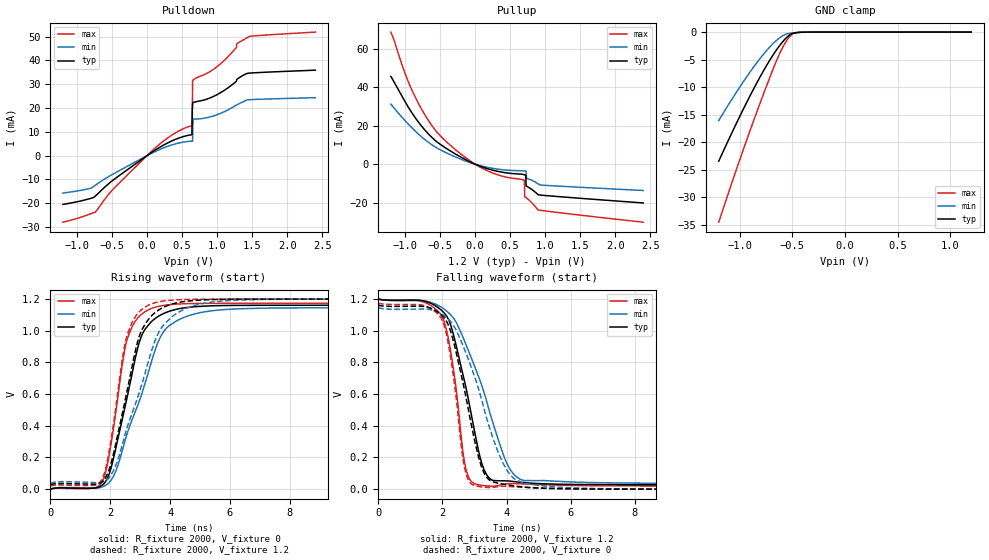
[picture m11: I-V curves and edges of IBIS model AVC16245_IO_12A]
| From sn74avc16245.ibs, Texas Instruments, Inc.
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[Model]   AVC16245_IO_12A
Model_type  I/O
Vinl = 0
Vinh = 1.2
Enable   Active-Low
Vref =   0
Rref =   2000
Cref =   30p
Vmeas =   0.6
| variable   typ   min   max
C_comp   6.68pF   6.18pF   7.38pF
| C_pullup   3.49pF   0.03pF   6.05pF
| C_pulldown   6.30pF   2.05pF   10.38pF
| C_tri-state   6.68pF   6.18pF   7.38pF
[Temperature Range]   40   100   -40
| Ambient temperature   25   85   -40
[Voltage range]   1.2   1.2   1.2
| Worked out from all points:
|   slope of the pulldown table from 0 to 0.18 V, typ, clamps not added: 51.7 ohm
|   slope of the pullup table from 0 to 0.18 V, typ, clamps not added: 75.9 ohm
|   GND clamp passes 1 mA (typ) near -0.56 V on its own axis
|   rising waveform, R_fixture 2000, V_fixture 0: 20-80 % time 818ps typ, 1.19ns min, 574ps max; typ from 0 V to 1.16 V
|   falling waveform, R_fixture 2000, V_fixture 1.2: 20-80 % time 749ps typ, 1.19ns min, 455ps max; typ from 1.2 V to 0.028 V
|   rising waveform, R_fixture 2000, V_fixture 1.2: 20-80 % time 816ps typ, 1.18ns min, 575ps max; typ from 0.028 V to 1.2 V
|   falling waveform, R_fixture 2000, V_fixture 0: 20-80 % time 741ps typ, 1.13ns min, 445ps max; typ from 1.16 V to 0 V
[GND Clamp]
| AVC16245_IO_12A
|   Voltage   I(typ)   I(min)   I(max)
-1.2V     -23.48mA   -16.09mA   -34.58mA
-1.055V   -17.52mA   -11.63mA   -26.28mA
-920mV    -12.26mA   -7.746mA   -18.87mA
-800mV    -7.914mA   -4.632mA   -12.58mA
-700mV    -4.663mA   -2.414mA   -7.551mA
-640mV    -2.948mA   -1.337mA   -4.735mA
-590mV    -1.713mA   -656.6uA   -2.719mA
-545mV    -820.2uA   -290.5uA   -1.288mA
-505mV    -294.5uA   -174.3uA   -438.8uA
-455mV    -91.21uA   -79.33uA   -93.44uA
-385mV    -13.73uA   -21.91uA   -7.311uA
1.2V      671.7pA    3.121nA    23.8pA
[Pulldown]
| AVC16245_IO_12A
|   Voltage   I(typ)   I(min)   I(max)
-1.2V     -20.49mA   -15.71mA   -27.96mA
-735mV    -16.93mA   -12.4mA    -23.63mA
-490mV    -10.42mA   -7.841mA   -14.3mA
105mV     2.117mA    1.578mA    2.919mA
640mV     8.777mA    6.078mA    12.49mA
645mV     19.09mA    6.084mA    12.56mA
650mV     22.11mA    6.1mA      31.26mA
655mV     22.27mA    14.99mA    31.78mA
1.02V     25.96mA    17.43mA    37.88mA
1.29V     32.23mA    21.49mA    47.14mA
1.46V     34.67mA    23.51mA    50.08mA
2.4V      35.9mA     24.35mA    51.89mA
[Pullup]
| AVC16245_IO_12A
|   Voltage   I(typ)   I(min)   I(max)
-1.2V     45.5mA     31.17mA    68.57mA
-950mV    29.56mA    20.73mA    42.76mA
-735mV    18.6mA     13.35mA    26.89mA
-175mV    3.153mA    2.205mA    4.536mA
230mV     -2.893mA   -2.023mA   -4.269mA
705mV     -5.502mA   -3.55mA    -8.484mA
710mV     -5.555mA   -3.566mA   -16.92mA
725mV     -5.74mA    -3.634mA   -17.28mA
730mV     -11.38mA   -3.665mA   -17.41mA
735mV     -11.47mA   -7.353mA   -17.54mA
900mV     -15.81mA   -10.2mA    -23.72mA
2.4V      -20.15mA   -13.67mA   -30.14mA
[Ramp]
| AVC16245_IO_12A
| variable   typ   min   max
dV/dt_r   0.70/8.23E-10   0.69/1.19E-09   0.70/5.77E-10
dV/dt_f   0.70/7.51E-10   0.70/1.19E-09   0.71/4.59E-10
R_load = 2000
[Rising Waveform]
| AVC16245_IO_12A
R_fixture =   2000
C_fixture =   0
L_fixture =   0
V_fixture =   0
V_fixture_min = 0
V_fixture_max = 0
|   Time   V(typ)   V(min)   V(max)
0s        24.7nV     138.2nV    665.8pV
1.51ns    7.743mV    6.93mV     9.912mV
1.845ns   47.28mV    24.35mV    105.5mV
2.18ns    251.3mV    110.4mV    473.7mV
2.605ns   614.7mV    372.8mV    967.2mV
3.08ns    981.3mV    617mV      1.109V
3.865ns   1.115V     1.014V     1.162V
4.995ns   1.154V     1.114V     1.172V
7.165ns   1.161V     1.143V     1.173V
50ns      1.161V     1.145V     1.173V
[Falling Waveform]
| AVC16245_IO_12A
R_fixture =   2000
C_fixture =   0
L_fixture =   0
V_fixture =   1.2
V_fixture_min = 1.2
V_fixture_max = 1.2
|   Time   V(typ)   V(min)   V(max)
0s        1.2V       1.2V       1.2V
1.35ns    1.19V      1.191V     1.185V
1.99ns    1.126V     1.146V     1.089V
2.285ns   1.018V     1.094V     836.7mV
2.74ns    636.1mV    910.6mV    122.6mV
3.27ns    137.7mV    627.6mV    22.9mV
3.53ns    59.43mV    447.8mV    18.77mV
4.005ns   52.17mV    164.8mV    33.91mV
4.58ns    40.67mV    53.88mV    32.26mV
50ns      27.74mV    36.95mV    20.19mV
[Rising Waveform]
| AVC16245_IO_12A
R_fixture =   2000
C_fixture =   0
L_fixture =   0
V_fixture =   1.2
V_fixture_min = 1.2
V_fixture_max = 1.2
|   Time   V(typ)   V(min)   V(max)
0s        27.75mV    36.95mV    20.19mV
1.525ns   31.67mV    40.61mV    27.06mV
1.83ns    67.56mV    51.42mV    116.6mV
2.18ns    281.7mV    146.8mV    507mV
2.615ns   665.9mV    417.7mV    997.7mV
3.065ns   1.008V     667.9mV    1.136V
3.845ns   1.154V     1.048V     1.189V
4.925ns   1.193V     1.165V     1.199V
6.99ns    1.2V       1.198V     1.2V
50ns      1.2V       1.2V       1.2V
[Falling Waveform]
| AVC16245_IO_12A
R_fixture =   2000
C_fixture =   0
L_fixture =   0
V_fixture =   0
V_fixture_min = 0
V_fixture_max = 0
|   Time   V(typ)   V(min)   V(max)
0s        1.161V     1.145V     1.173V
1.405ns   1.154V     1.137V     1.16V
1.97ns    1.099V     1.106V     1.075V
2.26ns    994.3mV    1.057V     826.8mV
2.705ns   610.6mV    874.1mV    121.1mV
3.24ns    129.9mV    552.1mV    13.41mV
3.72ns    38.36mV    242.6mV    15.69mV
4.15ns    23.09mV    83.17mV    15.88mV
5.765ns   2.566mV    10.71mV    3.773mV
50ns      -3.853uV   -6.011uV   -2.161uV
